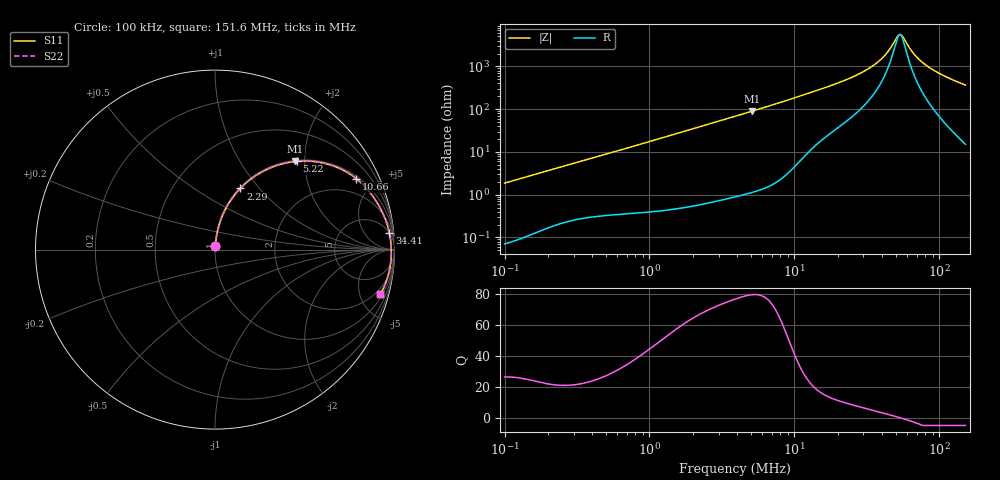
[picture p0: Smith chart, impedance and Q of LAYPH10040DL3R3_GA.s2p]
! LAYPH10040DL3R3_GA  S-PARAMETER MODEL  ( General Type )
! Model Generated by TAIYO YUDEN Corporation (http://www.ty-top.com)
! Version 1.0
! TAIYO YUDEN Control No. 180920NI43SB-FBB
! Copyright(c) 2018 TAIYO YUDEN CO.,LTD. All Rights Reserved.
! Product Description (link to TY-COMPAS)
! https://ds.yuden.co.jp/TYCOMPAS/or/detail?pn=LAYPH10040DL3R3NGA&u=M
! Products Name : Inductors
! Characteristics :
!  Inductance : 3.3 uH , SRF(min) : -Hz , DC Resistance(max) : 0.017 Ohm
!  Rated Current : Saturation :6.6 A , Temp Rise : 2.9 A (25 degC)
!  Case Size : 10.1 x 10.0 / 0.398 x 0.394 [mm/inch] , Thickness : 4 / 0.157 [mm/inch]
!  (Conditions: Temperature = 25 degC , DC Bias Current/Voltage = 0A / 0V)
! External Node Assignments :
!  1  o---GGG---o  2
! GND o---------o GND
! Frequency Range : 0.1MHz  -  151.640846MHz  [ 402 STEP ]
# MHz S RI R 50
! Freq[MHz].  S11 Real  S11 Imag  S21 Real  S21 Imag  S12 Real  S12 Imag  S22 Real  S22 Imag
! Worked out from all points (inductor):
!   401 points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, 100 kHz to 151.6 MHz, reference 50 ohm
!   read as one part in series: L = 2.95 uH near 103.7 kHz
!   highest Q = 79.5 at 5.125 MHz (marker M1), where L = 2.79 uH
!   self-resonance near 53.4 MHz
!   S11 on the Smith chart (normalised r, x): 100 kHz: 1.00, +0.04; 2.29 MHz: 1.01, +0.80; 5.22 MHz: 1.02, +1.83; 10.66 MHz: 1.11, +3.93; 34.41 MHz: 5, +20; 151.6 MHz: 1.30, -7.33
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0.1  0.00105 0.0186  0.9989 -0.0186  0.9989 -0.0186  0.00105 0.0186
0.341025  0.00643 0.0604  0.9936 -0.0604  0.9936 -0.0604  0.00643 0.0604
0.659265  0.0166 0.1134  0.9834 -0.1134  0.9834 -0.1134  0.0166 0.1134
1.162983  0.0433 0.1935  0.9567 -0.1935  0.9567 -0.1935  0.0433 0.1935
2.289807  0.1411 0.3408  0.8589 -0.3408  0.8589 -0.3408  0.1411 0.3408
3.894109  0.3187 0.4595  0.6813 -0.4595  0.6813 -0.4595  0.3187 0.4595
5.124939  0.4482 0.4911  0.5518 -0.4911  0.5518 -0.4911  0.4482 0.4911
5.219642  0.4574 0.4919  0.5426 -0.4919  0.5426 -0.4919  0.4574 0.4919
7.25734  0.6243 0.4773  0.3757 -0.4773  0.3757 -0.4773  0.6243 0.4773
10.66032  0.7881 0.3946  0.2119 -0.3946  0.2119 -0.3946  0.7881 0.3946
13.2799  0.8522 0.3319  0.1478 -0.3319  0.1478 -0.3319  0.8522 0.3319
23.42654  0.9441 0.1813  0.0559 -0.1813  0.0559 -0.1813  0.9441 0.1813
34.41129  0.9716 0.0931  0.0284 -0.0931  0.0284 -0.0931  0.9716 0.0931
39.83981  0.9772 0.0617  0.0228 -0.0617  0.0228 -0.0617  0.9772 0.0617
45.28783  0.9804 0.0349  0.0196 -0.0349  0.0196 -0.0349  0.9804 0.0349
51.48086  0.9822 0.00827  0.0178 -0.00827  0.0178 -0.00827  0.9822 0.00827
54.38786  0.9825 -0.00314  0.0175 0.00314  0.0175 0.00314  0.9825 -0.00314
56.41648  0.9825 -0.0108  0.0175 0.0108  0.0175 0.0108  0.9825 -0.0108
66.52339  0.9814 -0.0455  0.0186 0.0455  0.0186 0.0455  0.9814 -0.0455
79.89043  0.977 -0.0855  0.023 0.0855  0.023 0.0855  0.977 -0.0855
105.1418  0.9628 -0.1504  0.0372 0.1504  0.0372 0.1504  0.9628 -0.1504
151.6408  0.9219 -0.2485  0.0781 0.2485  0.0781 0.2485  0.9219 -0.2485
